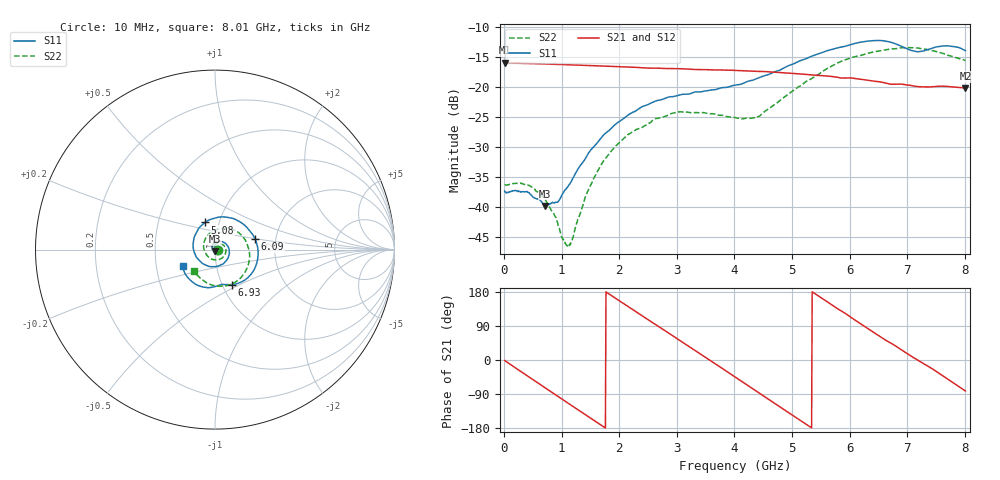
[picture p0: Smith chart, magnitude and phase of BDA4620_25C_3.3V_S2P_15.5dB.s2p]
!Agilent Technologies,E5071B,MY42404982,A.09.10
!Date: Wed May 06 08:51:54 2026
!Data & Calibration Information:
!Freq	S11:SOLT2(ON)	S21:SOLT2(ON)	S12:SOLT2(ON)	S22:SOLT2(ON)
# Hz S RI R 50
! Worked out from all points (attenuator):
!   801 points, 10 MHz to 8.01 GHz, reference 50 ohm
!   highest |S21| = -15.92 dB at 10 MHz (marker M1); lowest = -20.2 dB at 8.01 GHz (marker M2)
!   lowest |S11| = -39.8 dB at 710 MHz (marker M3), VSWR 1.02, Z = 50 - j1.02 ohm
!   |S11| at or under -10 dB: start of sweep to end of sweep
!   |S22| runs from -46.5 to -13.4 dB; largest |S21 - S12| = 0.00068
!   S11 on the Smith chart (normalised r, x): 10 MHz: 1.03, -0.00; 5.08 GHz: 0.86, +0.27; 6.09 GHz: 1.56, +0.19; 6.93 GHz: 1.11, -0.45; 8.01 GHz: 0.69, -0.13
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1e7  0.0136 -0.000844  0.16 -0.00338  0.16 -0.00346  0.0154 -0.000646
4.3e8  0.00951 -0.00925  0.1125 -0.1103  0.1125 -0.1106  0.0137 -0.0067
7.1e8  -0.000305 -0.0102  0.0455 -0.1494  0.0454 -0.1496  0.00733 -0.00899
9.4e8  -0.00956 -0.00578  -0.0174 -0.1538  -0.0176 -0.1542  0.000561 -0.00701
1.11e9  -0.0148 0.00142  -0.0621 -0.1409  -0.0622 -0.1411  -0.0041 -0.00261
1.18e9  -0.0158 0.00571  -0.0786 -0.1316  -0.0789 -0.1318  -0.00523 -4.56e-05
1.35e9  -0.0165 0.0162  -0.1134 -0.1018  -0.1135 -0.102  -0.00722 0.00658
1.58e9  -0.00991 0.0312  -0.1429 -0.0484  -0.1431 -0.0486  -0.00567 0.0173
1.89e9  0.0119 0.0454  -0.1455 0.0322  -0.1456 0.0323  0.00538 0.0301
2.68e9  0.0779 0.00428  0.00346 0.1439  0.00366 0.144  0.0519 0.0187
3.4e9  0.0351 -0.0842  0.1346 0.0404  0.1348 0.0404  0.0459 -0.0406
4.01e9  -0.071 -0.0759  0.0981 -0.0971  0.0982 -0.0973  -0.0196 -0.0525
4.41e9  -0.1191 -0.00264  0.0117 -0.1347  0.0115 -0.1351  -0.0553 -0.0123
5.08e9  -0.0556 0.151  -0.1155 -0.059  -0.1158 -0.059  -0.0235 0.0958
5.35e9  0.0206 0.1808  -0.1265 0.000284  -0.1267 0.000265  0.0275 0.1155
6.09e9  0.224 0.0576  -0.0318 0.1139  -0.0319 0.1141  0.1746 0.0421
6.39e9  0.2362 -0.0606  0.028 0.1095  0.028 0.1095  0.193 -0.0317
6.68e9  0.1745 -0.1636  0.0722 0.0786  0.0725 0.0787  0.1767 -0.1074
6.93e9  0.0921 -0.1953  0.0966 0.0425  0.0969 0.0426  0.137 -0.1636
7.19e9  0.0354 -0.1943  0.101 -0.00162  0.1014 -0.00158  0.0686 -0.2004
7.58e9  -0.0705 -0.2077  0.0806 -0.0625  0.081 -0.0625  -0.0366 -0.19
8.01e9  -0.1793 -0.0919  0.0141 -0.097  0.0142 -0.0972  -0.118 -0.1175
